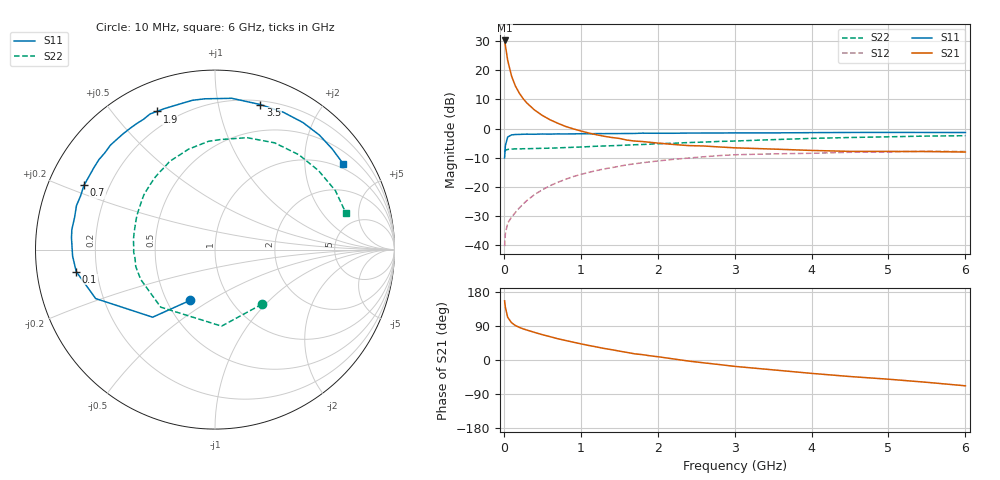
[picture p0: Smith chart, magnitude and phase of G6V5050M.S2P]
! SIEMENS Small Signal Semiconductors
! BFG193
! Si NPN RF Bipolar Junction Transistor in SOT223
! VCE = 0.5 V  IC = 50 mA
! Common Emitter S-Parameters:  August  1996
# GHz  S  MA  R  50
!  f  S11  S21  S12  S22
! GHz  MAG  ANG  MAG  ANG  MAG  ANG  MAG  ANG
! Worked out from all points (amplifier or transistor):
!   36 points, 10 MHz to 6 GHz, reference 50 ohm
!   highest |S21| = 30.2 dB at 10 MHz (marker M1)
!   |S21| within 3 dB of that: start of sweep to 27.7 MHz
!   unconditionally stable (mu >= 1): start of sweep to 14.75 MHz; 131.4 MHz to end of sweep
!   at 250 MHz: K = 1.22, MAG = 15.3 dB, |S12| = -25.8 dB
!   at 1.4 GHz: K = 1.26, MAG = 2.1 dB, |S12| = -13.4 dB
!   at 6 GHz: K = 1.07, MAG = -1.7 dB, |S12| = -7.8 dB
!   S11 on the Smith chart (normalised r, x): 10 MHz: 0.65, -0.41; 100 MHz: 0.12, -0.08; 700 MHz: 0.11, +0.23; 1.9 GHz: 0.13, +0.66; 3.5 GHz: 0.23, +1.33; 6 GHz: 0.85, +3.09
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0.01  0.3148 -116.1  32.47 156.1  0.0097 66.0  0.4015 -49.2
0.02  0.5125 -132.7  26.75 138.8  0.016 54.0  0.428 -85.1
0.05  0.7187 -157.7  14.82 112.7  0.0241 41.8  0.4408 -133.3
0.1  0.7828 -171.0  7.98 98.4  0.0304 45.6  0.4461 -158.1
0.15  0.7942 -177.4  5.394 91.0  0.0366 50.1  0.4515 -167.9
0.2  0.7974 178.3  4.082 86.2  0.0437 53.9  0.4483 -173.7
0.25  0.8024 175.2  3.274 82.3  0.051 56.4  0.4534 -178.3
0.3  0.8054 172.0  2.75 79.0  0.0587 57.9  0.4528 178.9
0.4  0.8025 167.2  2.083 72.8  0.0744 59.4  0.458 172.9
0.5  0.8097 162.4  1.686 66.9  0.0897 58.6  0.4605 168.1
0.6  0.8065 158.3  1.422 61.6  0.1054 57.6  0.4633 164.1
0.7  0.8132 153.8  1.241 56.2  0.1204 56.1  0.4684 160.4
0.9  0.8145 146.1  0.995 47.1  0.1509 51.7  0.4795 152.5
1.1  0.8168 138.9  0.845 38.5  0.1777 47.0  0.4921 145.8
1.6  0.8267 121.6  0.638 20.0  0.2399 33.8  0.5235 129.4
1.9  0.8349 112.8  0.584 11.1  0.27 26.2  0.5426 120.1
2.2  0.8343 104.1  0.537 3.0  0.2979 17.8  0.5619 110.9
3  0.8482 83.7  0.47 -16.8  0.3572 -2.6  0.6138 87.2
3.5  0.8468 72.6  0.447 -26.0  0.37 -15.9  0.6487 74.0
4.5  0.861 55.3  0.408 -43.6  0.3939 -34.5  0.7057 48.4
5.5  0.8609 40.7  0.405 -58.9  0.4128 -55.3  0.7469 26.1
6  0.8597 33.7  0.398 -68.1  0.4063 -67.2  0.7571 15.6
